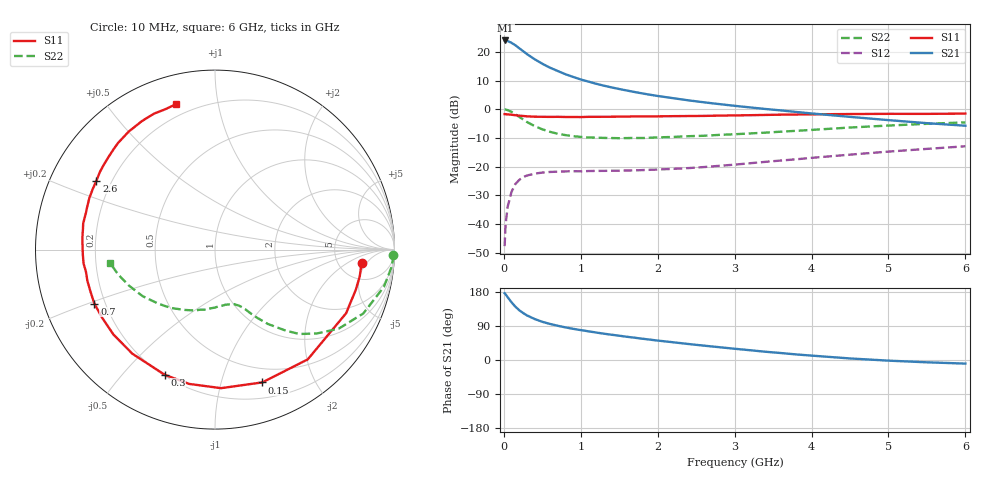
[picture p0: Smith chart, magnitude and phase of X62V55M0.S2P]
! SIEMENS Small Signal Semiconductors
! BFP193W
! Si NPN RF Bipolar Junction Transistor in SOT343
! VCE = 2.5 V  IC = 5 mA
! Common Emitter S-Parameters:  April 1994
# GHz  S  MA  R  50
!  f  S11  S21  S12  S22
! GHz  MAG  ANG  MAG  ANG  MAG  ANG  MAG  ANG
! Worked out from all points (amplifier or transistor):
!   40 points, 10 MHz to 6 GHz, reference 50 ohm
!   highest |S21| = 24.0 dB at 20 MHz (marker M1)
!   |S21| within 3 dB of that: start of sweep to 214.6 MHz
!   unconditionally stable (mu >= 1): 1.687 GHz to 4.371 GHz
!   at 200 MHz: K = 0.14, MSG = 23.0 dB, |S12| = -24.7 dB
!   at 1.5 GHz: K = 0.93, MSG = 14.2 dB, |S12| = -21.4 dB
!   at 6 GHz: K = 0.92, MSG = 3.6 dB, |S12| = -12.9 dB
!   lowest NFmin = 1.20 dB at 450 MHz
!   S11 on the Smith chart (normalised r, x): 10 MHz: 8.38, -3.81; 150 MHz: 0.35, -1.36; 300 MHz: 0.20, -0.66; 700 MHz: 0.16, -0.21; 2.6 GHz: 0.14, +0.26; 6 GHz: 0.14, +0.76
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0.01  0.8204 -5.2  15.71 176.2  0.0041 87.6  0.9944 -1.7
0.02  0.82 -10.6  15.78 174.1  0.0082 84.0  0.9902 -5.2
0.05  0.812 -25.9  15.42 165.5  0.02 77.1  0.9633 -12.5
0.1  0.8007 -49.8  14.35 152.3  0.0363 65.3  0.8997 -23.3
0.15  0.7854 -70.4  13.01 140.7  0.0497 55.6  0.8179 -32.6
0.2  0.7727 -87.5  11.56 131.4  0.0585 47.8  0.7348 -39.5
0.25  0.762 -100.9  10.3 124.0  0.0655 42.0  0.665 -45.0
0.3  0.7515 -111.9  9.145 117.7  0.0698 37.2  0.599 -48.9
0.4  0.7405 -128.4  7.439 108.2  0.0754 30.8  0.508 -54.6
0.5  0.7376 -140.1  6.204 100.8  0.0786 27.2  0.4463 -58.3
0.6  0.7346 -149.0  5.294 95.1  0.0806 24.4  0.4038 -61.0
0.7  0.7365 -155.9  4.633 90.4  0.0816 23.0  0.3735 -63.0
0.9  0.7319 -166.3  3.653 82.3  0.0831 21.3  0.3389 -66.9
1.1  0.7363 -173.9  3.028 75.7  0.0836 21.0  0.3218 -70.7
1.3  0.738 179.4  2.572 69.5  0.0842 21.8  0.3159 -74.9
1.6  0.7444 171.3  2.115 61.3  0.0855 24.0  0.3138 -80.9
2.2  0.7567 157.7  1.557 46.8  0.0913 30.3  0.3284 -94.4
2.6  0.7642 149.8  1.32 37.9  0.0981 34.8  0.3443 -103.7
3.2  0.7862 139.0  1.075 25.8  0.1143 39.4  0.3782 -117.4
4.5  0.8237 119.6  0.735 4.1  0.1615 41.3  0.4794 -147.2
5.5  0.8293 109.8  0.571 -6.1  0.2035 37.7  0.5562 -165.4
6  0.8382 105.2  0.515 -9.5  0.2259 35.3  0.5896 -172.7
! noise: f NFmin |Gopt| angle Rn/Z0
0.45  1.2  0.26  102  0.14
0.9  1.25  0.38  145  0.12
1.8  2.05  0.56  -161  0.12
